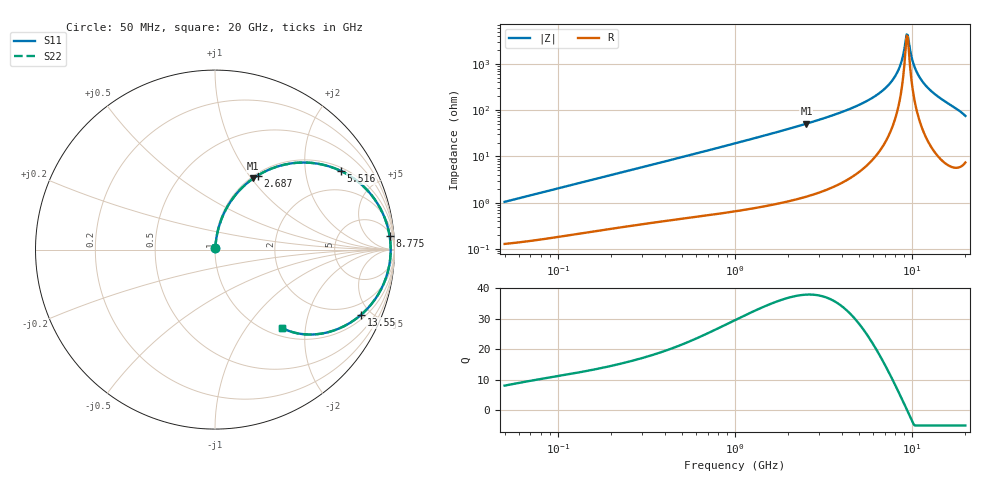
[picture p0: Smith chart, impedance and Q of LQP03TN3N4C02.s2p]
!Murata Part Number: LQP03TN3N4C02
!These Parameters are Measured in Series Mode Connection
!  o--[Z]--o
!Port1  Port2
!  o-------o
!Freq. Start=50[MHz] Stop=20[GHz], 401[Steps]
# Hz S RI R 50
!Freq.(Hz) S11(Real) S11(Imag) S21(Real) S21(Imag) S12(Real) S12(Imag) S22(Real) S22(Imag)
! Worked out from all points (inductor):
!   401 points, 50 MHz to 20 GHz, reference 50 ohm
!   read as one part in series: L = 3.27 nH near 51.52 MHz
!   highest Q = 38 at 2.531 GHz (marker M1), where L = 3.22 nH
!   self-resonance near 9.317 GHz
!   S11 on the Smith chart (normalised r, x): 50 MHz: 1.00, +0.02; 2.687 GHz: 1.03, +1.10; 5.516 GHz: 1.12, +3.13; 8.775 GHz: 8, +24; 13.55 GHz: 1.24, -4.36; 20 GHz: 1.15, -1.50
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5e7  0.00138 0.0103  0.9986 -0.0103  0.9986 -0.0103  0.00138 0.0103
1.364002e8  0.00291 0.0272  0.9971 -0.0272  0.9971 -0.0272  0.00291 0.0272
3.721004e8  0.00894 0.0713  0.9911 -0.0713  0.9911 -0.0713  0.00894 0.0713
1e9  0.0413 0.1827  0.9587 -0.1827  0.9587 -0.1827  0.0413 0.1827
2.531158e9  0.2137 0.397  0.7863 -0.397  0.7863 -0.397  0.2137 0.397
2.687447e9  0.2372 0.4124  0.7628 -0.4124  0.7628 -0.4124  0.2372 0.4124
2.728004e9  0.2434 0.4162  0.7566 -0.4162  0.7566 -0.4162  0.2434 0.4162
4.087748e9  0.4706 0.4846  0.5294 -0.4846  0.5294 -0.4846  0.4706 0.4846
5.515528e9  0.7028 0.4376  0.2972 -0.4376  0.2972 -0.4376  0.7028 0.4376
6.503449e9  0.8298 0.3497  0.1702 -0.3497  0.1702 -0.3497  0.8298 0.3497
7.442007e9  0.9144 0.2414  0.0856 -0.2414  0.0856 -0.2414  0.9144 0.2414
8.264682e9  0.9588 0.1382  0.0412 -0.1382  0.0412 -0.1382  0.9588 0.1382
8.774992e9  0.9733 0.0739  0.0267 -0.0739  0.0267 -0.0739  0.9733 0.0739
9.178299e9  0.9783 0.0242  0.0217 -0.0242  0.0217 -0.0242  0.9783 0.0242
9.457416e9  0.9789 -0.00936  0.0211 0.00936  0.0211 0.00936  0.9789 -0.00936
9.600142e9  0.9782 -0.0262  0.0218 0.0262  0.0218 0.0262  0.9782 -0.0262
1.019291e10  0.9699 -0.093  0.0301 0.093  0.0301 0.093  0.9699 -0.093
1.082228e10  0.9524 -0.1581  0.0476 0.1581  0.0476 0.1581  0.9524 -0.1581
1.183995e10  0.9096 -0.2493  0.0904 0.2493  0.0904 0.2493  0.9096 -0.2493
1.354865e10  0.8136 -0.3633  0.1864 0.3633  0.1864 0.3633  0.8136 -0.3633
1.670968e10  0.6078 -0.4652  0.3922 0.4652  0.3922 0.4652  0.6078 -0.4652
2e10  0.3742 -0.437  0.6258 0.437  0.6258 0.437  0.3742 -0.437
